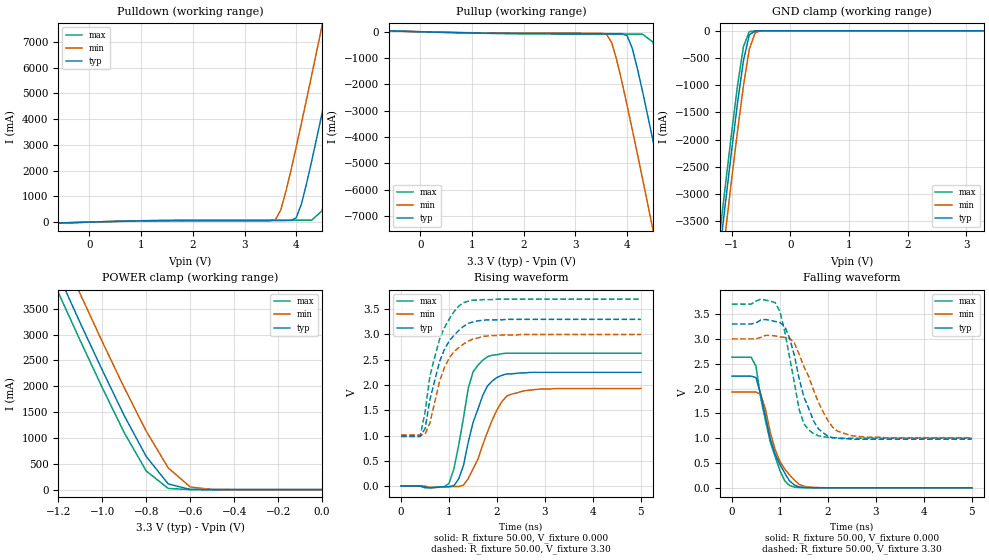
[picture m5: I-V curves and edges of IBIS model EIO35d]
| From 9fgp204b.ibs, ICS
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|   Model EIO35d
[Model]   EIO35d
Model_type   I/O
Polarity   Non-Inverting
Enable   Active-High
Vinl =   0.80V
Vinh =   2.00V
Vmeas =   1.50V
C_comp   3.40pF   2.85pF   3.95pF
[Temperature Range]   27.00   70.00   0.000
[Voltage Range]   3.30V   3.00V   3.70V
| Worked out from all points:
|   slope of the pulldown table from 0 to 0.495 V, typ, clamps not added: 18 ohm
|   slope of the pullup table from 0 to 0.495 V, typ, clamps not added: 20.5 ohm
|   GND clamp passes 1 mA (typ) near -0.54 V on its own axis
|   POWER clamp passes 1 mA (typ) near -0.53 V on its own axis
|   rising waveform, R_fixture 50.00, V_fixture 0.000: 20-80 % time 397ps typ, 497ps min, 312ps max; typ from 0 V to 2.25 V
|   rising waveform, R_fixture 50.00, V_fixture 3.30: 20-80 % time 427ps typ, 417ps min, 408ps max; typ from 0.98 V to 3.3 V
|   falling waveform, R_fixture 50.00, V_fixture 0.000: 20-80 % time 394ps typ, 388ps min, 384ps max; typ from 2.25 V to 0 V
|   falling waveform, R_fixture 50.00, V_fixture 3.30: 20-80 % time 410ps typ, 537ps min, 316ps max; typ from 3.3 V to 0.98 V
[Pulldown]
| voltage   I(typ)   I(min)   I(max)
|  -3.30   0.000A   -0.16A   10.00mA
|  -3.10   0.000A   0.000A   0.000A
|  -2.90   10.00mA   0.000A   0.000A
|  -2.70   0.000A   0.000A   0.000A
|  -2.50   0.000A   0.000A   0.000A
|  -2.30   0.000A   0.000A   0.000A
|  -2.10   0.000A   0.000A   0.000A
|  -1.90   0.000A   0.000A   0.000A
|  -1.70   -2.00mA   -2.00mA   -1.00mA
|  -1.50   -2.00mA   -2.00mA   -1.00mA
|  -1.00   -5.00mA   -4.00mA   -6.00mA
|  -0.90   -7.00mA   -5.00mA   -9.00mA
|  -0.80   -13.80mA   -8.00mA   -21.20mA
|  -0.70   -31.45mA   -16.10mA   -40.91mA
-600mV    -34.97mA   -28.05mA   -38.05mA
3.6V      62.07mA    100mA      76.52mA
3.7V      62.12mA    470mA      76.57mA
4V        170mA      2.92A      76.76mA
4.1V      700mA      3.84A      76.83mA
4.3V      2.38A      5.72A      77.42mA
4.5V      4.23A      7.64A      440mA
4.7V      6.14A      9.58A      2.05A
4.9V      8.07A      11.53A     3.9A
5.1V      10.02A     13.49A     5.81A
5.3V      11.98A     15.45A     7.75A
6.6V      24.84A     28.32A     20.56A
[Pullup]
| voltage   I(typ)   I(min)   I(max)
|  -3.30   10.00mA   0.000A   0.000A
|  -3.10   0.000A   10.00mA   0.000A
|  -2.90   10.00mA   0.000A   0.000A
|  -2.70   0.000A   0.000A   0.000A
|  -2.50   0.000A   0.000A   0.000A
|  -2.30   0.000A   0.000A   0.000A
|  -2.10   0.000A   0.000A   0.000A
|  -1.90   10.00mA   0.000A   0.000A
|  -1.70   2.00mA   2.00mA   1.00mA
|  -1.50   2.00mA   2.00mA   2.00mA
|  -1.00   5.00mA   4.00mA   6.00mA
|  -0.90   6.00mA   4.00mA   8.00mA
|  -0.80   12.10mA   7.00mA   18.80mA
|  -0.70   27.70mA   13.70mA   39.07mA
-600mV    32.95mA    25.43mA    36.49mA
3.6V      -71.57mA   -90.38mA   -90.02mA
3.8V      -72.16mA   -1.07A     -90.65mA
4V        -150mA     -2.79A     -91.23mA
4.1V      -620mA     -3.71A     -91.5mA
4.3V      -2.27A     -5.59A     -92.46mA
4.5V      -4.12A     -7.51A     -390mA
4.7V      -6.03A     -9.45A     -1.96A
4.9V      -7.97A     -11.4A     -3.81A
5.1V      -9.92A     -13.36A    -5.72A
5.3V      -11.88A    -15.33A    -7.66A
6.6V      -24.75A    -28.22A    -20.48A
[GND_clamp]
| voltage   I(typ)   I(min)   I(max)
-3.3V     -24.57A    -25.08A    -24.27A
-1.2V     -4.03A     -4.57A     -3.7A
-1.1V     -3.1A      -3.64A     -2.77A
-1V       -2.19A     -2.72A     -1.86A
-900mV    -1.32A     -1.84A     -1A
-800mV    -550mA     -1.01A     -290mA
-700mV    -72.95mA   -340mA     -14.76mA
-600mV    -2.33mA    -32.82mA   -460uA
-500mV    -100uA     -1.33mA    -46.85uA
3.3V      35.65uA    26.86uA    51.23uA
[POWER_clamp]
| voltage   I(typ)   I(min)   I(max)
-3.3V     24.7A      25.22A     24.38A
-1.2V     4.16A      4.71A      3.81A
-1.1V     3.22A      3.78A      2.88A
-1V       2.31A      2.86A      1.97A
-900mV    1.43A      1.97A      1.1A
-800mV    640mA      1.13A      360mA
-700mV    110mA      420mA      22.45mA
-600mV    3.45mA     51.18mA    440uA
-500mV    120uA      2.16mA     57.35uA
0V        35.65nA    24.07nA    51.27nA
[Ramp]
| variable   typ   min   max
dV/dt_r   1.35/0.39n   1.16/0.48n   1.58/0.32n
dV/dt_f   1.39/0.40n   1.19/0.50n   1.62/0.34n
R_load = 50.00
[Rising Waveform]
R_fixture = 50.00
V_fixture = 0.000
V_fixture_min = 0.000
V_fixture_max = 0.000
| time   V(typ)   V(min)   V(max)
0s        420uV      330uV      520uV
1ns       -13.5mV    -11.49mV   56.51mV
1.2ns     140mV      -9.04mV    810mV
1.3ns     410mV      18.31mV    1.35V
1.4ns     870mV      150mV      1.94V
1.5ns     1.26V      340mV      2.26V
1.8ns     1.98V      1.07V      2.56V
2.1ns     2.19V      1.67V      2.62V
2.3ns     2.22V      1.82V      2.63V
5ns       2.25V      1.93V      2.63V
[Rising Waveform]
R_fixture = 50.00
V_fixture = 3.30
V_fixture_min = 3.00
V_fixture_max = 3.70
| time   V(typ)   V(min)   V(max)
0s        980mV      1.01V      1V
400ps     980mV      1.01V      1V
500ps     1.14V      1.03V      1.47V
600ps     1.71V      1.25V      2.18V
800ps     2.46V      2.07V      2.9V
1ns       2.87V      2.53V      3.3V
1.3ns     3.16V      2.81V      3.63V
1.5ns     3.25V      2.91V      3.68V
1.9ns     3.29V      2.98V      3.69V
5ns       3.3V       3V         3.7V
[Falling Waveform]
R_fixture = 50.00
V_fixture = 0.000
V_fixture_min = 0.000
V_fixture_max = 0.000
| time   V(typ)   V(min)   V(max)
0s        2.25V      1.93V      2.63V
400ps     2.25V      1.93V      2.63V
500ps     2.22V      1.93V      2.45V
600ps     1.88V      1.88V      1.8V
800ps     980mV      1.11V      920mV
1ns       470mV      530mV      350mV
1.2ns     140mV      260mV      48.6mV
1.4ns     18.98mV    70.38mV    7.25mV
1.7ns     3.41mV     9.94mV     2.06mV
5ns       480uV      380uV      600uV
[Falling Waveform]
R_fixture = 50.00
V_fixture = 3.30
V_fixture_min = 3.00
V_fixture_max = 3.70
| time   V(typ)   V(min)   V(max)
0s        3.3V       3V         3.7V
900ps     3.35V      3.06V      3.73V
1.1ns     3.25V      3.03V      3.15V
1.3ns     2.67V      2.92V      2.12V
1.4ns     2.2V       2.69V      1.58V
1.5ns     1.83V      2.44V      1.29V
1.7ns     1.35V      1.97V      1.09V
2.1ns     1.01V      1.22V      1.01V
2.5ns     980mV      1.05V      1V
5ns       980mV      1.01V      1V
